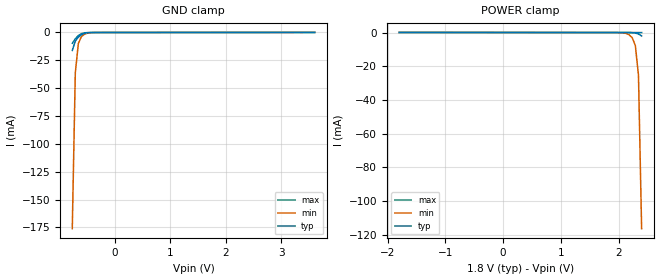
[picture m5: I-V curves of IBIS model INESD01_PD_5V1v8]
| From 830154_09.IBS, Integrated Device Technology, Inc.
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| 2.50909e+00   -3.85956e-03   -5.33565e-01   -2.23540e-04
| 2.56364e+00   -8.05444e-03   -8.01228e-01   -6.86326e-04
| 2.61818e+00   -2.98680e-02   -1.06902e+00   -1.68547e-03
| 2.67273e+00   -1.92881e-01   -1.33693e+00   -3.29196e-03
| 2.72727e+00   -5.14252e-01   -1.60492e+00   -5.42233e-03
| 2.78182e+00   -8.35766e-01   -1.87300e+00   -8.22540e-03
| 2.83636e+00   -1.15740e+00   -2.14114e+00   -1.59052e-02
| 2.89091e+00   -1.47913e+00   -2.40934e+00   -9.34784e-02
| 2.94545e+00   -1.80094e+00   -2.67759e+00   -4.79844e-01
| 3.00000e+00   -2.12280e+00   -2.94587e+00   -8.90786e-01
| 3.05455e+00   -2.44472e+00   -3.21420e+00   -1.30181e+00
| 3.10909e+00   -2.76669e+00   -3.48256e+00   -1.71290e+00
| 3.16364e+00   -3.08869e+00   -3.75094e+00   -2.12404e+00
| 3.21818e+00   -3.41071e+00   -4.01935e+00   -2.53522e+00
| 3.27273e+00   -3.73276e+00   -4.28777e+00   -2.94643e+00
| 3.32727e+00   -4.05484e+00   -4.55622e+00   -3.35766e+00
| 3.38182e+00   -4.37692e+00   -4.82467e+00   -3.76890e+00
| 3.43636e+00   -4.69902e+00   -5.09314e+00   -4.18016e+00
| 3.49091e+00   -5.02114e+00   -5.36162e+00   -4.59142e+00
| 3.54545e+00   -5.34325e+00   -5.63011e+00   -5.00269e+00
| 3.60000e+00   -5.66538e+00   -5.89861e+00   -5.41396e+00
[Model] INESD01_PD_5V1v8
Model_type   Input
Polarity   Non-Inverting
Vinl = 0.5775V
Vinh = 1.2675V
|   typ   min   max
C_comp   2pF   1.5pF   2.5pF
|   typ   min   max
[Voltage range]   1.8V   1.65V   1.95V
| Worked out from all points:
|   GND clamp passes 1 mA (typ) near -0.55 V on its own axis
[GND_clamp]
|Voltage   I (typ)   I (min)   I (max)
|Note, modeling breaks down at 250mA and above.  This is well beyond the functional   |
|operating range of the device.  Should this scenario occur, catastrophic failure and   |
|possible damage to the device and/or board is of higher concern than the I-V curve   |
|behavior.  The IBIS checker will flag currents in excess of 10A with warnings.  Lines   |
|with currents in excess of 0.35 A have been commented out.  The points still remain|
|available to the user if the user desires to use them.   |
|-1.80000e+00   -1.13307e+01   -1.03205e+01   -1.30899e+01
|-1.74545e+00   -1.06865e+01   -9.78355e+00   -1.22674e+01
|-1.69091e+00   -1.00423e+01   -9.24663e+00   -1.14448e+01
|-1.63636e+00   -9.39803e+00   -8.70974e+00   -1.06223e+01
|-1.58182e+00   -8.75383e+00   -8.17288e+00   -9.79974e+00
|-1.52727e+00   -8.10966e+00   -7.63606e+00   -8.97720e+00
|-1.47273e+00   -7.46552e+00   -7.09928e+00   -8.15468e+00
|-1.41818e+00   -6.82142e+00   -6.56256e+00   -7.33217e+00
|-1.36364e+00   -6.17736e+00   -6.02589e+00   -6.50969e+00
|-1.30909e+00   -5.53337e+00   -5.48929e+00   -5.68725e+00
|-1.25455e+00   -4.88944e+00   -4.95278e+00   -4.86485e+00
|-1.20000e+00   -4.24560e+00   -4.41636e+00   -4.04251e+00
|-1.14545e+00   -3.60187e+00   -3.88005e+00   -3.22025e+00
|-1.09091e+00   -2.95826e+00   -3.34386e+00   -2.39810e+00
|-1.03636e+00   -2.31480e+00   -2.80783e+00   -1.57609e+00
|-9.81818e-01   -1.67153e+00   -2.27196e+00   -7.54252e-01
|-9.27273e-01   -1.02850e+00   -1.73632e+00   -1.06690e-01
|-8.72727e-01   -3.85760e-01   -1.20093e+00   -2.51898e-02
|-8.18182e-01   -5.97340e-02   -6.65821e-01   -1.48150e-02
-763.6mV  -16.11mA   -176mA     -9.691mA
-709.1mV  -7.715mA   -36.19mA   -5.674mA
-654.5mV  -4.204mA   -9.999mA   -2.752mA
-600mV    -2.058mA   -3.793mA   -1.05mA
-545.5mV  -843.7uA   -1.609mA   -322.5uA
-490.9mV  -291.7uA   -643.9uA   -86.86uA
-327.3mV  -10.69uA   -28.26uA   -5.255uA
3.6V      70.14uA    87.71uA    54.35uA
[Power_clamp]
|Voltage   I (typ)   I (min)   I (max)
|Note, modeling breaks down at 250mA and above.  This is well beyond the functional   |
|operating range of the device.  Should this scenario occur, catastrophic failure and   |
|possible damage to the device and/or board is of higher concern than the I-V curve   |
|behavior.  The IBIS checker will flag currents in excess of 10A with warnings.  Lines   |
|with currents in excess of 0.35 A have been commented out.  The points still remain|
|available to the user if the user desires to use them.   |
-1.8V     70.14uA    84.05uA    56.61uA
1.964V    -3.208uA   -22.23uA   -205.9nA
2.073V    -6.106uA   -179.5uA   -1.853uA
2.182V    -27.8uA    -1.291mA   -3.505uA
2.236V    -90.3uA    -3.056mA   -4.382uA
2.291V    -291.7uA   -7.663mA   -5.686uA
2.345V    -843.7uA   -25.37mA   -10.13uA
2.4V      -2.058mA   -116.4mA   -31.6uA
